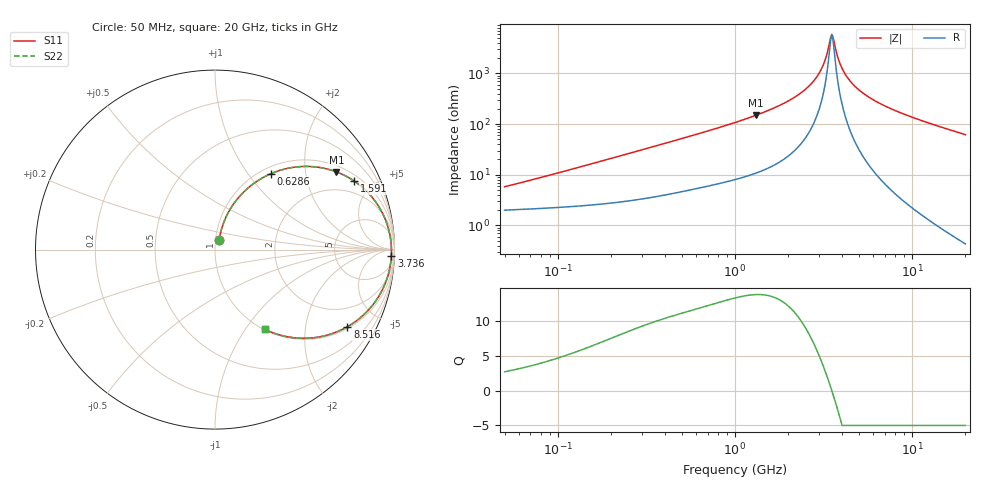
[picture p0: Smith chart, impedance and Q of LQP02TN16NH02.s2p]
!Murata Part Number: LQP02TN16NH02
!These Parameters are Measured in Series Mode Connection
!  o--[Z]--o
!Port1  Port2
!  o-------o
!Freq. Start=50[MHz] Stop=20[GHz], 401[Steps]
# Hz S RI R 50
!Freq.(Hz) S11(Real) S11(Imag) S21(Real) S21(Imag) S12(Real) S12(Imag) S22(Real) S22(Imag)
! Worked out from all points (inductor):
!   401 points, 50 MHz to 20 GHz, reference 50 ohm
!   read as one part in series: L = 17.1 nH near 57.22 MHz
!   highest Q = 13.8 at 1.309 GHz (marker M1), where L = 18 nH
!   self-resonance near 3.519 GHz
!   S11 on the Smith chart (normalised r, x): 50 MHz: 1.04, +0.11; 628.6 MHz: 1.11, +1.30; 1.591 GHz: 1.29, +3.88; 3.736 GHz: 23, -47; 8.516 GHz: 1.07, -3.39; 20 GHz: 1.01, -1.24
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5e7  0.0224 0.0521  0.9776 -0.0521  0.9776 -0.0521  0.0224 0.0521
1.364002e8  0.0425 0.134  0.9575 -0.134  0.9575 -0.134  0.0425 0.134
3.721004e8  0.1523 0.3133  0.8477 -0.3133  0.8477 -0.3133  0.1523 0.3133
6.285508e8  0.3122 0.4232  0.6878 -0.4232  0.6878 -0.4232  0.3122 0.4232
1e9  0.5323 0.4629  0.4677 -0.4629  0.4677 -0.4629  0.5323 0.4629
1.309461e9  0.6764 0.4331  0.3236 -0.4331  0.3236 -0.4331  0.6764 0.4331
1.590961e9  0.7746 0.3827  0.2254 -0.3827  0.2254 -0.3827  0.7746 0.3827
2.179053e9  0.9017 0.2564  0.0983 -0.2564  0.0983 -0.2564  0.9017 0.2564
2.728004e9  0.9585 0.1422  0.0415 -0.1422  0.0415 -0.1422  0.9585 0.1422
3.121702e9  0.977 0.0681  0.023 -0.0681  0.023 -0.0681  0.977 0.0681
3.265178e9  0.9804 0.0429  0.0196 -0.0429  0.0196 -0.0429  0.9804 0.0429
3.466789e9  0.983 0.00905  0.017 -0.00905  0.017 -0.00905  0.983 0.00905
3.572216e9  0.9833 -0.00795  0.0167 0.00795  0.0167 0.00795  0.9833 -0.00795
3.736399e9  0.9827 -0.0335  0.0173 0.0335  0.0173 0.0335  0.9827 -0.0335
3.908127e9  0.9807 -0.059  0.0193 0.059  0.0193 0.059  0.9807 -0.059
4.087748e9  0.9774 -0.0845  0.0226 0.0845  0.0226 0.0845  0.9774 -0.0845
4.677679e9  0.9591 -0.1597  0.0409 0.1597  0.0409 0.1597  0.9591 -0.1597
5.683258e9  0.911 -0.2626  0.089 0.2626  0.089 0.2626  0.911 -0.2626
7.442007e9  0.805 -0.3835  0.195 0.3835  0.195 0.3835  0.805 -0.3835
8.516016e9  0.7377 -0.4297  0.2623 0.4297  0.2623 0.4297  0.7377 -0.4297
1.276073e10  0.5075 -0.4941  0.4925 0.4941  0.4925 0.4941  0.5075 -0.4941
2e10  0.2774 -0.4443  0.7226 0.4443  0.7226 0.4443  0.2774 -0.4443
